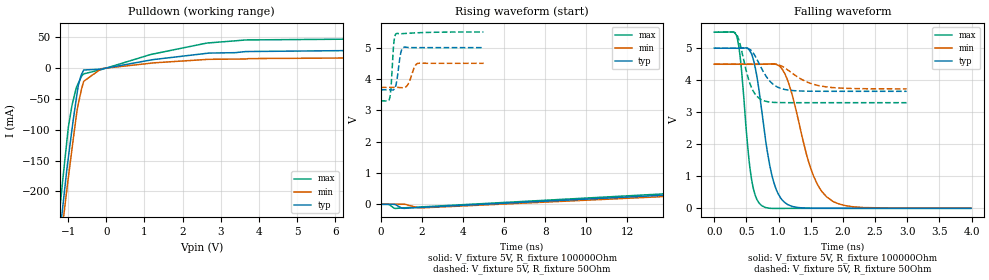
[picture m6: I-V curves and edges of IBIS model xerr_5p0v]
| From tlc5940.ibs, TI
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|   xerr_5p0v Model
[Model]   xerr_5p0v
Model_type   Open_drain
Polarity   Inverting
Vmeas = 1.65
Vref = 2.5
Cref = 15pF
Rref = 100000
|   typ   min   max
|   (nom PVT)   (Fast PVT)   (slow PVT)
|Average
C_comp   1.058e-12   1.048e-12   1.063e-12
|ON state : BUFFER OUTPUT TURNED LOW
|C_comp   1.150e-12   1.136e-12   1.155e-12
|OFF state: BUFFER in HIGH IMPEDANCE
|C_comp   9.669e-13   9.601e-13   9.711e-13
| Where nom  PVT is Nominal Process, 5V, 65C
|   Fast PVT is Strong Process,  5.5V, -40C
|   Slow PVT is Weak Process,   4.5V, 125C
[Voltage Range]   5   4.5   5.5
|Ambient Temperature   25   85   -40
|Junction Temperature
[Temperature Range]   65   125   -40
[Pullup Reference]   5   4.5   5.5
[Pulldown Reference]   0   0   0
[Power Clamp Reference]   5   4.5   5.5
[GND Clamp Reference]   0   0   0
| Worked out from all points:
|   slope of the pulldown table from 0 to 0.75 V, typ, clamps not added: 89 ohm
|   falling waveform, V_fixture 5V, R_fixture 100000Ohm: 20-80 % time 228ps typ, 364ps min, 146ps max; typ from 5 V to 0.005 V
|   rising waveform, V_fixture 5V, R_fixture 100000Ohm: 20-80 % time 141ns typ, 140ns min, 143ns max; typ from 0.004 V to 5 V
|   rising waveform, V_fixture 5V, R_fixture 50Ohm: 20-80 % time 168ps typ, 250ps min, 126ps max; typ from 3.65 V to 5 V
|   falling waveform, V_fixture 5V, R_fixture 50Ohm: 20-80 % time 245ps typ, 401ps min, 177ps max; typ from 5 V to 3.66 V
[Pulldown]
|   Voltage   I(typ)   I(min)   I(max)
-5V       -2.653A    -2.51A     -2.89A
-1.276V   -302mA     -326.1mA   -266.1mA
-1.166V   -239.8mA   -266.8mA   -197.8mA
-1.139V   -224.6mA   -252.5mA   -181.1mA
-1.036V   -166.4mA   -198.7mA   -120.5mA
-897mV    -99.09mA   -130.9mA   -60.33mA
-730mV    -27.39mA   -57.45mA   -24.37mA
-590mV    -3.112mA   -21.39mA   -9.379mA
-130mV    -1.67mA    -1.032mA   -2.443mA
2.672V    24.18mA    14.17mA    40.77mA
7.952V    29.34mA    17.03mA    47.74mA
10V       38.13mA    22.87mA    63.58mA
[Ramp]
R_load = 100000
|   typ   min   max
dV/dt_r   2.99758/1.40818e-07   2.69644/1.40292e-07   3.29841/1.43093e-07
dV/dt_f   2.99709/2.27939e-10   2.69548/3.62844e-10   3.29802/1.45806e-10
[Falling Waveform]
V_fixture = 5V
V_fixture_min = 4.5V
V_fixture_max = 5.5V
R_fixture = 100000Ohm
|   Time   V(typ)   V(min)   V(max)
0s        5V         4.5V       5.5V
350ps     4.999V     4.5V       5.37V
410ps     5.001V     4.5V       4.598V
570ps     4.862V     4.499V     1.041V
730ps     3.174V     4.5V       101mV
870ps     1.274V     4.509V     4.556mV
1.04ns    305.5mV    4.388V     1.612mV
1.53ns    8.809mV    1.084V     4.008mV
1.84ns    6.528mV    227.5mV    3.741mV
3.99ns    4.791mV    7.441mV    3.289mV
[Rising Waveform]
V_fixture = 5V
V_fixture_min = 4.5V
V_fixture_max = 5.5V
R_fixture = 100000Ohm
|   Time   V(typ)   V(min)   V(max)
0s        3.882mV    5.765mV    2.546mV
710ps     -10.3mV    5.757mV    -130mV
1.98ns    -95.67mV   -111.2mV   -79.32mV
72.51ns   2.139V     1.928V     2.266V
124.7ns   3.286V     2.959V     3.553V
183.2ns   4.077V     3.673V     4.447V
247.4ns   4.546V     4.094V     4.981V
326ns     4.814V     4.333V     5.286V
437.7ns   4.948V     4.453V     5.44V
900ns     5V         4.5V       5.5V
[Rising Waveform]
V_fixture = 5V
V_fixture_min = 4.5V
V_fixture_max = 5.5V
R_fixture = 50Ohm
|   Time   V(typ)   V(min)   V(max)
0s        3.655V     3.731V     3.3V
440ps     3.655V     3.731V     3.426V
500ps     3.651V     3.731V     3.812V
630ps     3.663V     3.731V     5.153V
730ps     3.799V     3.731V     5.439V
950ps     4.782V     3.725V     5.444V
1.13ns    5.015V     3.726V     5.449V
1.33ns    5.005V     3.842V     5.458V
1.79ns    5V         4.496V     5.474V
5ns       5V         4.5V       5.499V
[Falling Waveform]
V_fixture = 5V
V_fixture_min = 4.5V
V_fixture_max = 5.5V
R_fixture = 50Ohm
|   Time   V(typ)   V(min)   V(max)
0s        5V         4.5V       5.5V
340ps     5V         4.5V       5.454V
400ps     5.001V     4.5V       5.132V
570ps     4.938V     4.5V       3.817V
770ps     4.243V     4.501V     3.363V
930ps     3.853V     4.503V     3.31V
1.17ns    3.689V     4.282V     3.301V
1.44ns    3.66V      3.947V     3.3V
1.75ns    3.656V     3.791V     3.3V
2.99ns    3.656V     3.731V     3.3V
